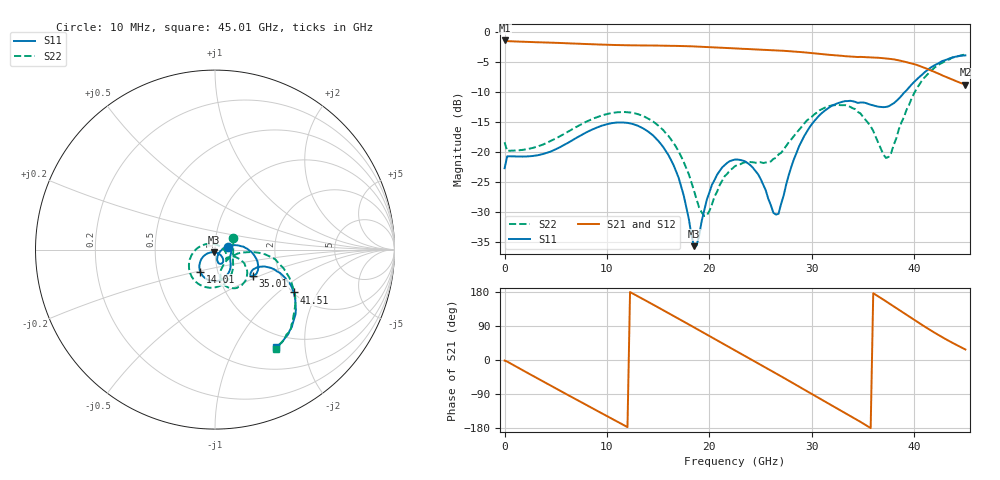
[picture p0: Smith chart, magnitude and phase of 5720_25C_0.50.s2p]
! Device:  ADRF5720
! Description: 0.5dB LSB GaAs MMIC 6-bit Digital Attenuator
! Frequency:  0.000009 -  40 GHz
! Ports:
!	RF1	= Port 1
!	RF2	= Port 2
! Vdd:  3.3 Volt
! Vss:  -3.3 Volt
! Control:  0/3.3 Volt
! State:  0.50 dB attenuation
! Data:  The device was measured using G-S-G Probes on a matrix board.
!  Data was collected using an calibrated 4 port network analyzer.
!  The reference plane for this measurement is at the launchers.
! Note:  Analog Devices supplies this data as a sample of measured data
!  for this product.  Your particular data for this product may vary.
!  Data was taken at 25 degrees C.
!  Analog Devices reserves the right to change this data at anytime.
# GHZ S DB R 45.0
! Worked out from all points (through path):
!   181 points, 10 MHz to 45.01 GHz, reference 45 ohm
!   highest |S21| = -1.36 dB at 10 MHz (marker M1); lowest = -8.7 dB at 45.01 GHz (marker M2)
!   group delay of S21, straight-line fit = 42.6 ps
!   lowest |S11| = -35.8 dB at 18.51 GHz (marker M3), VSWR 1.03, Z = 44.5 - j1.35 ohm
!   |S11| at or under -10 dB: start of sweep to 39.09 GHz
!   |S22| runs from -30.7 to -3.7 dB; largest |S21 - S12| = 0.0011
!   S11 on the Smith chart (normalised r, x): 10 MHz: 1.15, +0.04; 14.01 GHz: 0.83, -0.21; 35.01 GHz: 1.45, -0.46; 41.51 GHz: 2.02, -1.28; 45.01 GHz: 0.80, -1.48
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0.01  -22.74 12.8  -1.36 -1.5  -1.36 -1.5  -18.40 32.6
2.01  -20.78 -18.0  -1.59 -30.5  -1.59 -30.5  -19.60 -17.3
4.26  -20.09 -31.9  -1.72 -63.8  -1.71 -63.8  -18.39 -33.4
7.76  -16.94 -54.8  -1.94 -115.3  -1.94 -115.3  -15.14 -61.9
11.01  -15.09 -88.3  -2.13 -162.6  -2.13 -162.5  -13.37 -97.6
14.01  -16.58 -123.3  -2.20 153.6  -2.20 153.6  -14.40 -136.7
15.26  -18.66 -137.2  -2.22 135.0  -2.22 135.1  -15.97 -154.5
17.01  -24.36 -152.1  -2.28 108.8  -2.28 108.8  -19.94 176.4
18.51  -35.78 -111.3  -2.36 86.1  -2.36 86.1  -26.50 137.2
19.76  -27.99 -44.7  -2.45 67.2  -2.45 67.2  -30.65 54.6
21.26  -22.60 -51.7  -2.58 44.5  -2.58 44.5  -24.81 -10.2
22.76  -21.29 -65.6  -2.71 21.9  -2.71 21.9  -22.20 -31.6
24.76  -23.74 -78.1  -2.88 -8.4  -2.87 -8.3  -21.76 -40.5
26.76  -30.36 -17.9  -3.05 -39.1  -3.04 -39.0  -20.44 -24.6
28.26  -21.24 14.5  -3.21 -62.4  -3.21 -62.4  -17.36 -20.4
30.26  -14.83 1.2  -3.51 -93.7  -3.51 -93.6  -13.72 -31.4
35.01  -11.74 -35.0  -4.13 -167.3  -4.14 -167.2  -14.14 -76.1
37.01  -12.52 -31.0  -4.33 159.1  -4.33 159.2  -20.48 -58.2
37.76  -12.12 -24.9  -4.47 146.1  -4.48 146.2  -20.20 -22.5
39.76  -8.73 -19.4  -5.21 110.5  -5.20 110.6  -11.04 -5.4
41.51  -6.03 -28.6  -6.28 80.2  -6.28 80.2  -6.67 -23.4
45.01  -3.86 -58.2  -8.74 27.7  -8.74 27.8  -3.72 -58.6
